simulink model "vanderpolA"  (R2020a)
settings: Solver=ode45  StartTime=0.0  StopTime=100  RelTol=1e-3  EnableMultiTasking=on

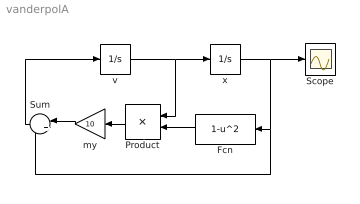
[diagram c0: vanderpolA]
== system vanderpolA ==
  note: .
  Fcn : Fcn  Expr=1-u^2
  Product : Product  InputSameDT=on  RndMeth=Zero  SaturateOnIntegerOverflow=on
  Scope : Scope
  Sum : Sum  Inputs=|+-  InputSameDT=on  SaturateOnIntegerOverflow=on
  my : Gain  Gain=10  SaturateOnIntegerOverflow=on
  v : Integrator
  x : Integrator  InitialCondition=0.5
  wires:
  x/1 -> Sum/2, Fcn/1, Scope/1
  v/1 -> Product/1, x/1
  Sum/1 -> v/1
  my/1 -> Sum/1
  Fcn/1 -> Product/2
  Product/1 -> my/1
